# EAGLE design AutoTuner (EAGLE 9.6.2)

## Sheet 1 of 4: mcu
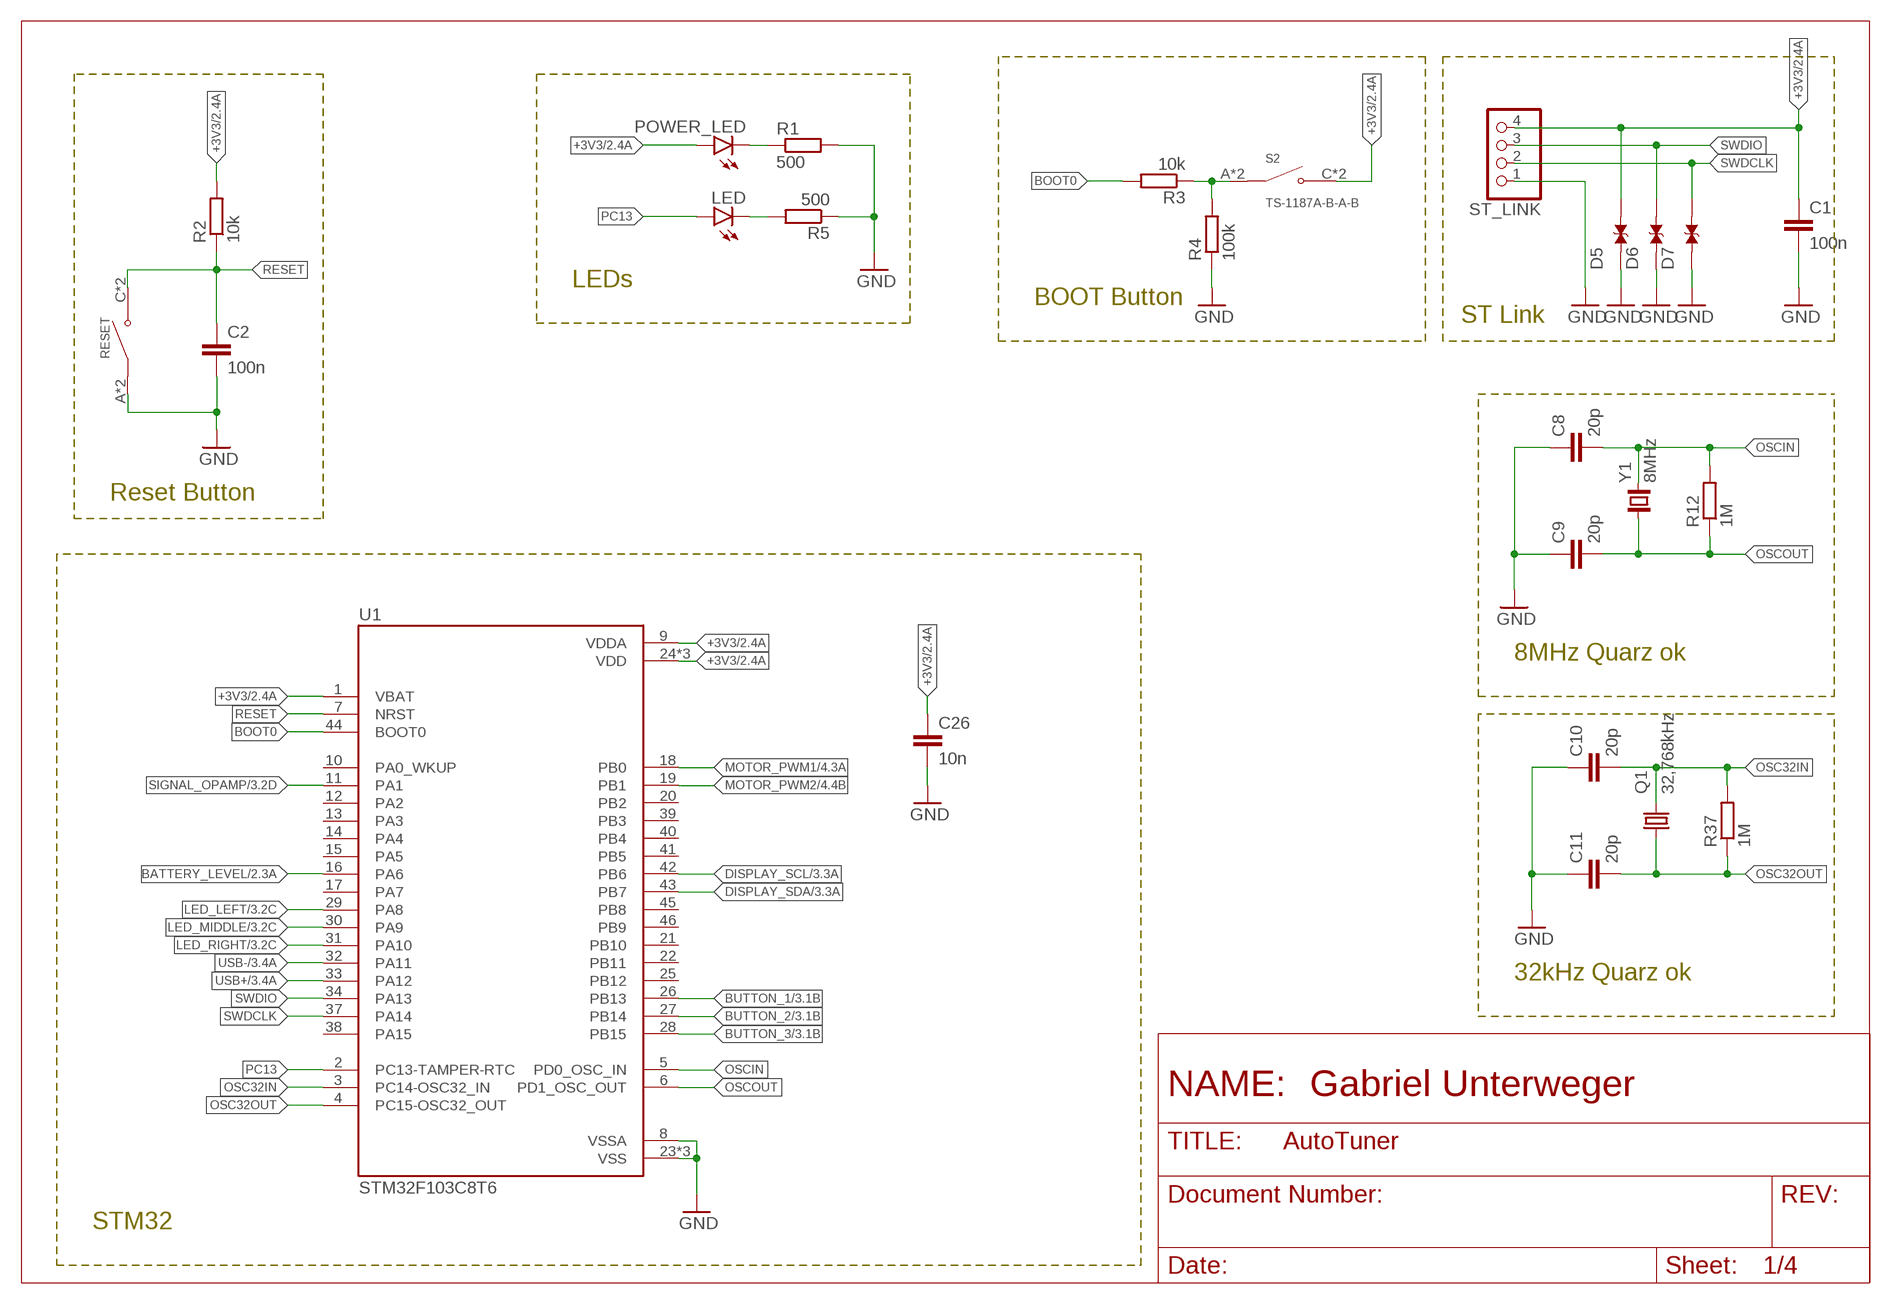
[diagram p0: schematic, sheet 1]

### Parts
C1  100n  C-EUC0805  [C0805]
C2  100n  C-EUC0805  [C0805]
C8  20p  C-EUC0805  [C0805]
C9  20p  C-EUC0805  [C0805]
C10  20p  C-EUC0805  [C0805]
C11  20p  C-EUC0805  [C0805]
C26  10n  C-EUC0805  [C0805]
D5  TESD5V0L1UC_RJG  [DIO_TESD5V0L1UC_RJG]
D6  TESD5V0L1UC_RJG  [DIO_TESD5V0L1UC_RJG]
D7  TESD5V0L1UC_RJG  [DIO_TESD5V0L1UC_RJG]
LED  LEDCHIPLED_0805  [CHIPLED_0805]
POWER_LED  LEDCHIPLED_0805  [CHIPLED_0805]
Q1  32,768kHz  KX-327-NHF  [3.2X1.5]
R1  500  R-EU_R0805  [R0805]
R2  10k  R-EU_R0805  [R0805]
R3  10k  R-EU_R0805  [R0805]
R4  100k  R-EU_R0805  [R0805]
R5  500  R-EU_R0805  [R0805]
R12  1M  R-EU_R0805  [R0805]
R37  1M  R-EU_R0805  [R0805]
RESET  TS-1187A-B-A-B  [SW_TS-1187A-B-A-B]
S2  TS-1187A-B-A-B  [SW_TS-1187A-B-A-B]
ST_LINK  PINHD-1X4  [1X04]
U1  STM32F103C8T6  [QFP50P900X900X160-48N]
Y1  8MHz  CRYSTAL_NX5032GA  [CRYSTAL_2-SMD-5X3]

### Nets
+3V3: C1.1 C26.1 D5.2 POWER_LED.A R2.2 S2.C(NO) S2.D(NO) ST_LINK.4 U1.1(VBAT) U1.9(VDDA) U1.24(VDD) U1.36(VDD) U1.48(VDD) ; also sheet 2,3,4
BATTERY_LEVEL: U1.16(PA6) ; also sheet 2
BOOT0: R3.2 U1.44(BOOT0)
BUTTON_1: U1.26(PB13) ; also sheet 3
BUTTON_2: U1.27(PB14) ; also sheet 3
BUTTON_3: U1.28(PB15) ; also sheet 3
DISPLAY_SCL: U1.42(PB6) ; also sheet 3
DISPLAY_SDA: U1.43(PB7) ; also sheet 3
GND: C1.2 C2.2 C8.1 C9.1 C10.1 C11.1 C26.2 D5.1 D6.1 D7.1 R1.2 R4.1 R5.1 RESET.A(COM) RESET.B(COM) ST_LINK.1 U1.8(VSSA) U1.23(VSS) U1.35(VSS) U1.47(VSS) ; also sheet 2,3,4
LED_LEFT: U1.29(PA8) ; also sheet 3
LED_MIDDLE: U1.30(PA9) ; also sheet 3
LED_RIGHT: U1.31(PA10) ; also sheet 3
MOTOR_PWM1: U1.18(PB0) ; also sheet 4
MOTOR_PWM2: U1.19(PB1) ; also sheet 4
N$2: LED.C R5.2
N$3: POWER_LED.C R1.1
N$5: R3.1 R4.2 S2.A(COM) S2.B(COM)
OSC32IN: C10.2 Q1.2 R37.2 U1.3(PC14-OSC32_IN)
OSC32OUT: C11.2 Q1.1 R37.1 U1.4(PC15-OSC32_OUT)
OSCIN: C8.2 R12.2 U1.5(PD0_OSC_IN) Y1.2
OSCOUT: C9.2 R12.1 U1.6(PD1_OSC_OUT) Y1.1
PC13: LED.A U1.2(PC13-TAMPER-RTC)
RESET: C2.1 R2.1 RESET.C(NO) RESET.D(NO) U1.7(NRST)
SIGNAL_OPAMP: U1.11(PA1) ; also sheet 3,4
SWDCLK: D7.2 ST_LINK.2 U1.37(PA14)
SWDIO: D6.2 ST_LINK.3 U1.34(PA13)
USB+: U1.33(PA12) ; also sheet 3
USB-: U1.32(PA11) ; also sheet 3
Unconnected: U1.10(PA0_WKUP) U1.12(PA2) U1.13(PA3) U1.14(PA4) U1.15(PA5) U1.17(PA7) U1.20(PB2) U1.21(PB10) U1.22(PB11) U1.25(PB12) U1.38(PA15) U1.39(PB3) U1.40(PB4) U1.41(PB5) U1.45(PB8) U1.46(PB9)

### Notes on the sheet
- LEDs
- BOOT Button
- ST Link
- Reset Button
- 8MHz Quarz ok
- 32kHz Quarz ok
- STM32

## Sheet 2 of 4: battery / voltage converter
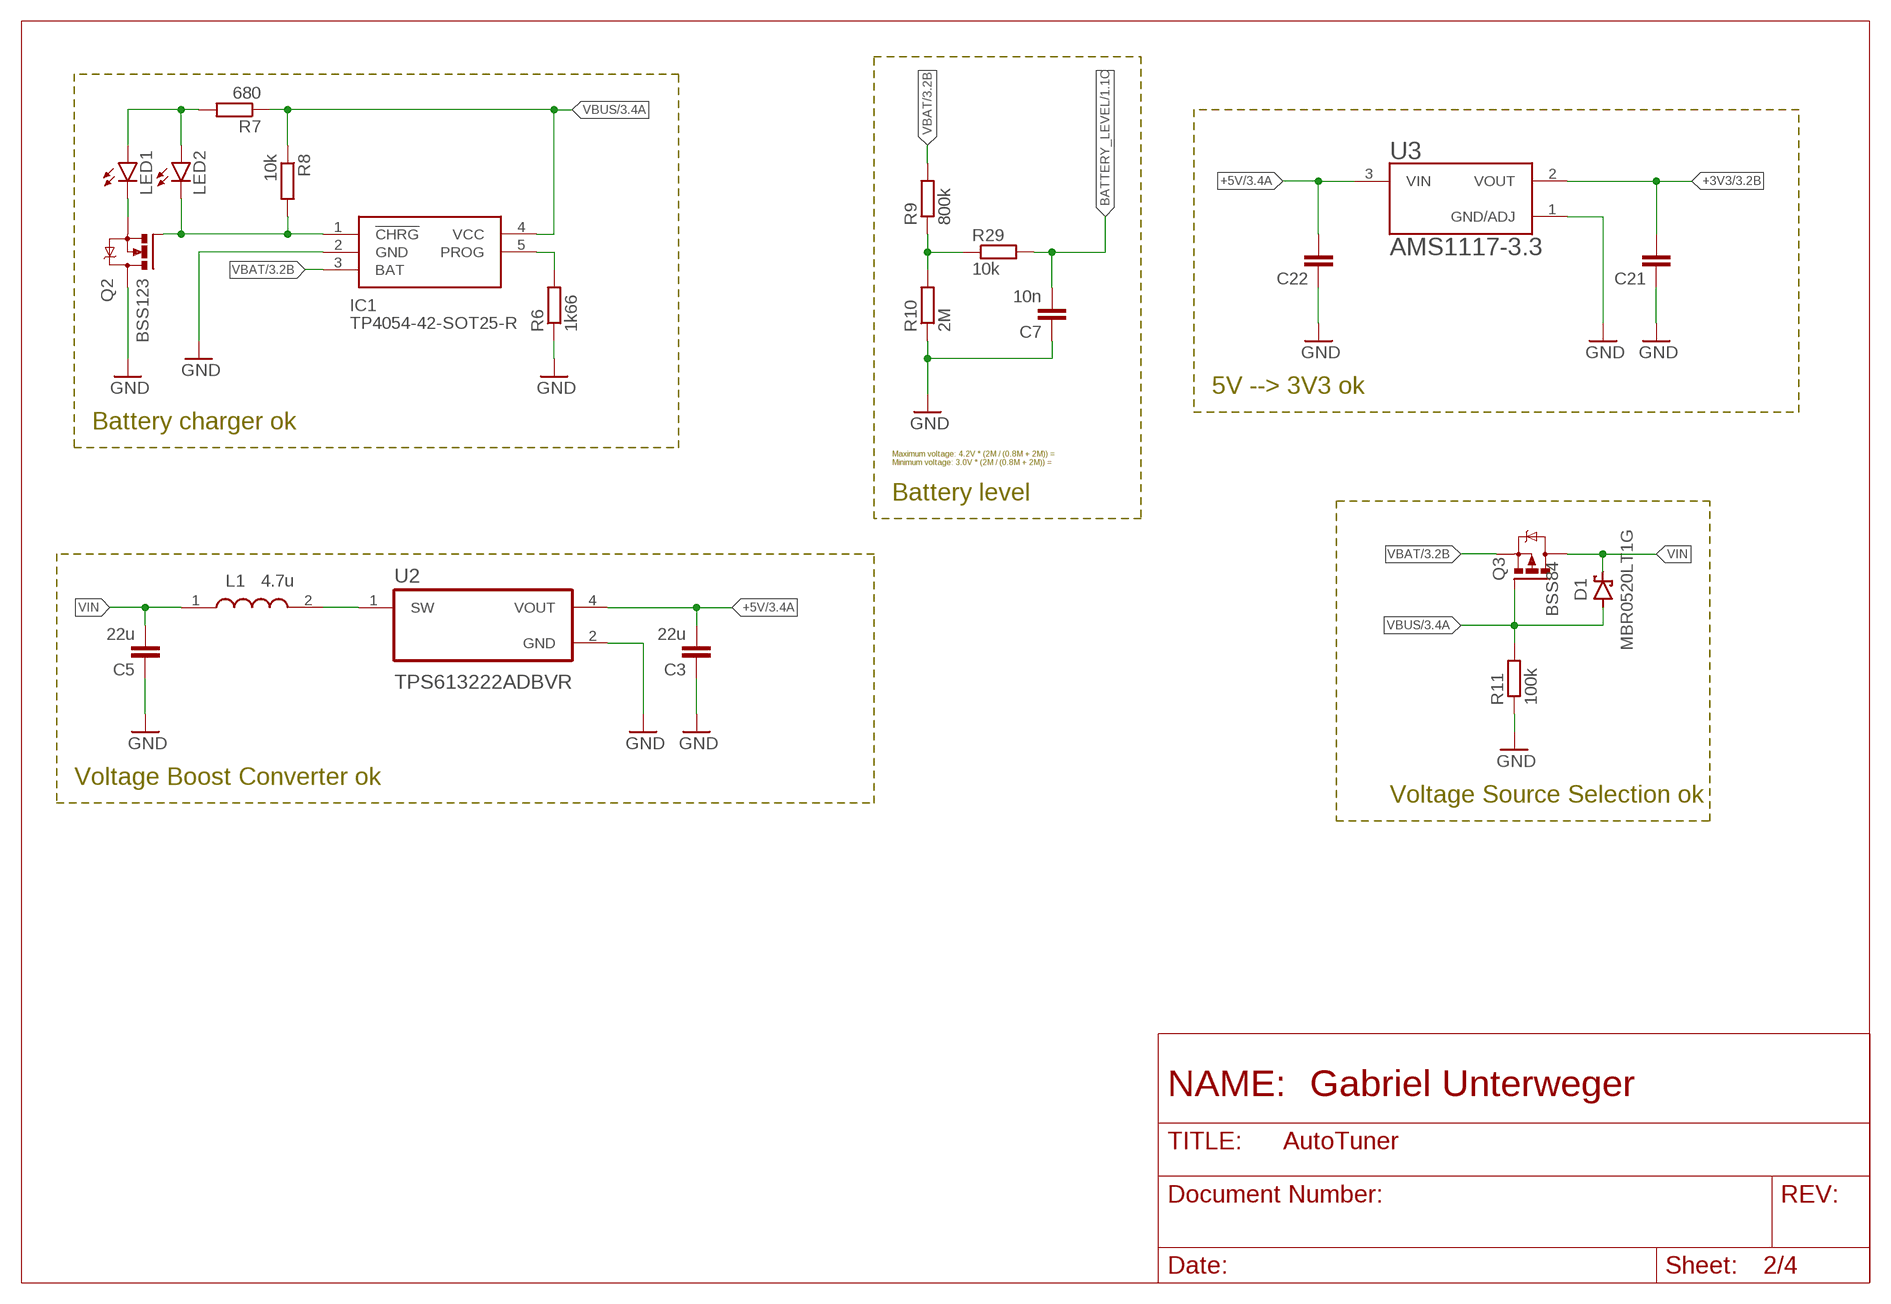
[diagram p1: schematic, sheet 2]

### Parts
C3  22u  C-EUC0805  [C0805]
C5  22u  C-EUC0805  [C0805]
C7  10n  C-EUC0805  [C0805]
C21  C-EUC0805  [C0805]
C22  C-EUC0805  [C0805]
D1  MBR0520LT1G  SCHOTTKY_MBR0520LT1GDO-219  [SODFL3718X115]
IC1  TP4054-42-SOT25-R  [SOT95P280X100-5N]
L1  4.7u  DFE252012P-4R7M=P2  [DFE2HCAH1R0MJ0L]
LED1  LEDCHIPLED_0805  [CHIPLED_0805]
LED2  LEDCHIPLED_0805  [CHIPLED_0805]
Q2  BSS123  NMOSFET_BSS123_SOT23-GSD  [SOT23]
Q3  BSS84  PMOSFET_BSS84_SOT23-GSD  [SOT23]
R6  1k66  R-EU_R0805  [R0805]
R7  680  R-EU_R0805  [R0805]
R8  10k  R-EU_R0805  [R0805]
R9  800k  R-EU_R0805  [R0805]
R10  2M  R-EU_R0805  [R0805]
R11  100k  R-EU_R0805  [R0805]
R29  10k  R-EU_R0805  [R0805]
U2  TPS613222ADBVR  [SOT95P280X145-5N]
U3  AMS1117-3.3  [SOT229P700X180-4N]

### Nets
+3V3: C21.2 U3.2(VOUT) ; also sheet 1,3,4
+5V: C3.2 C22.2 U2.4(VOUT) U3.3(VIN) ; also sheet 3
BATTERY_LEVEL: C7.2 R29.2 ; also sheet 1
GND: C3.1 C5.1 C7.1 C21.1 C22.1 IC1.2(GND) Q2.3(D) R6.1 R10.1 R11.1 U2.2(GND) U3.1(GND/ADJ) ; also sheet 1,3,4
N$1: L1.2 U2.1(SW)
N$4: R9.1 R10.2 R29.1
N$8: IC1.5(PROG) R6.2
N$9: IC1.1(!CHRG) LED2.C Q2.1(G) R8.2
N$11: LED1.A LED2.A R7.2
N$12: LED1.C Q2.2(S)
VBAT: IC1.3(BAT) Q3.2(S) R9.2 ; also sheet 3,4
VBUS: D1.2(A) IC1.4(VCC) Q3.1(G) R7.1 R8.1 R11.2 ; also sheet 3
VIN: C5.2 D1.1(C) L1.1 Q3.3(D)

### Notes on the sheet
- 5V --> 3V3 ok
- Battery charger ok
- Maximum voltage: 4.2V * (2M / (0.8M + 2M)) =
  Minimum voltage: 3.0V * (2M / (0.8M + 2M)) =
- Battery level
- Voltage Boost Converter ok
- Voltage Source Selection ok

## Sheet 3 of 4: I/O
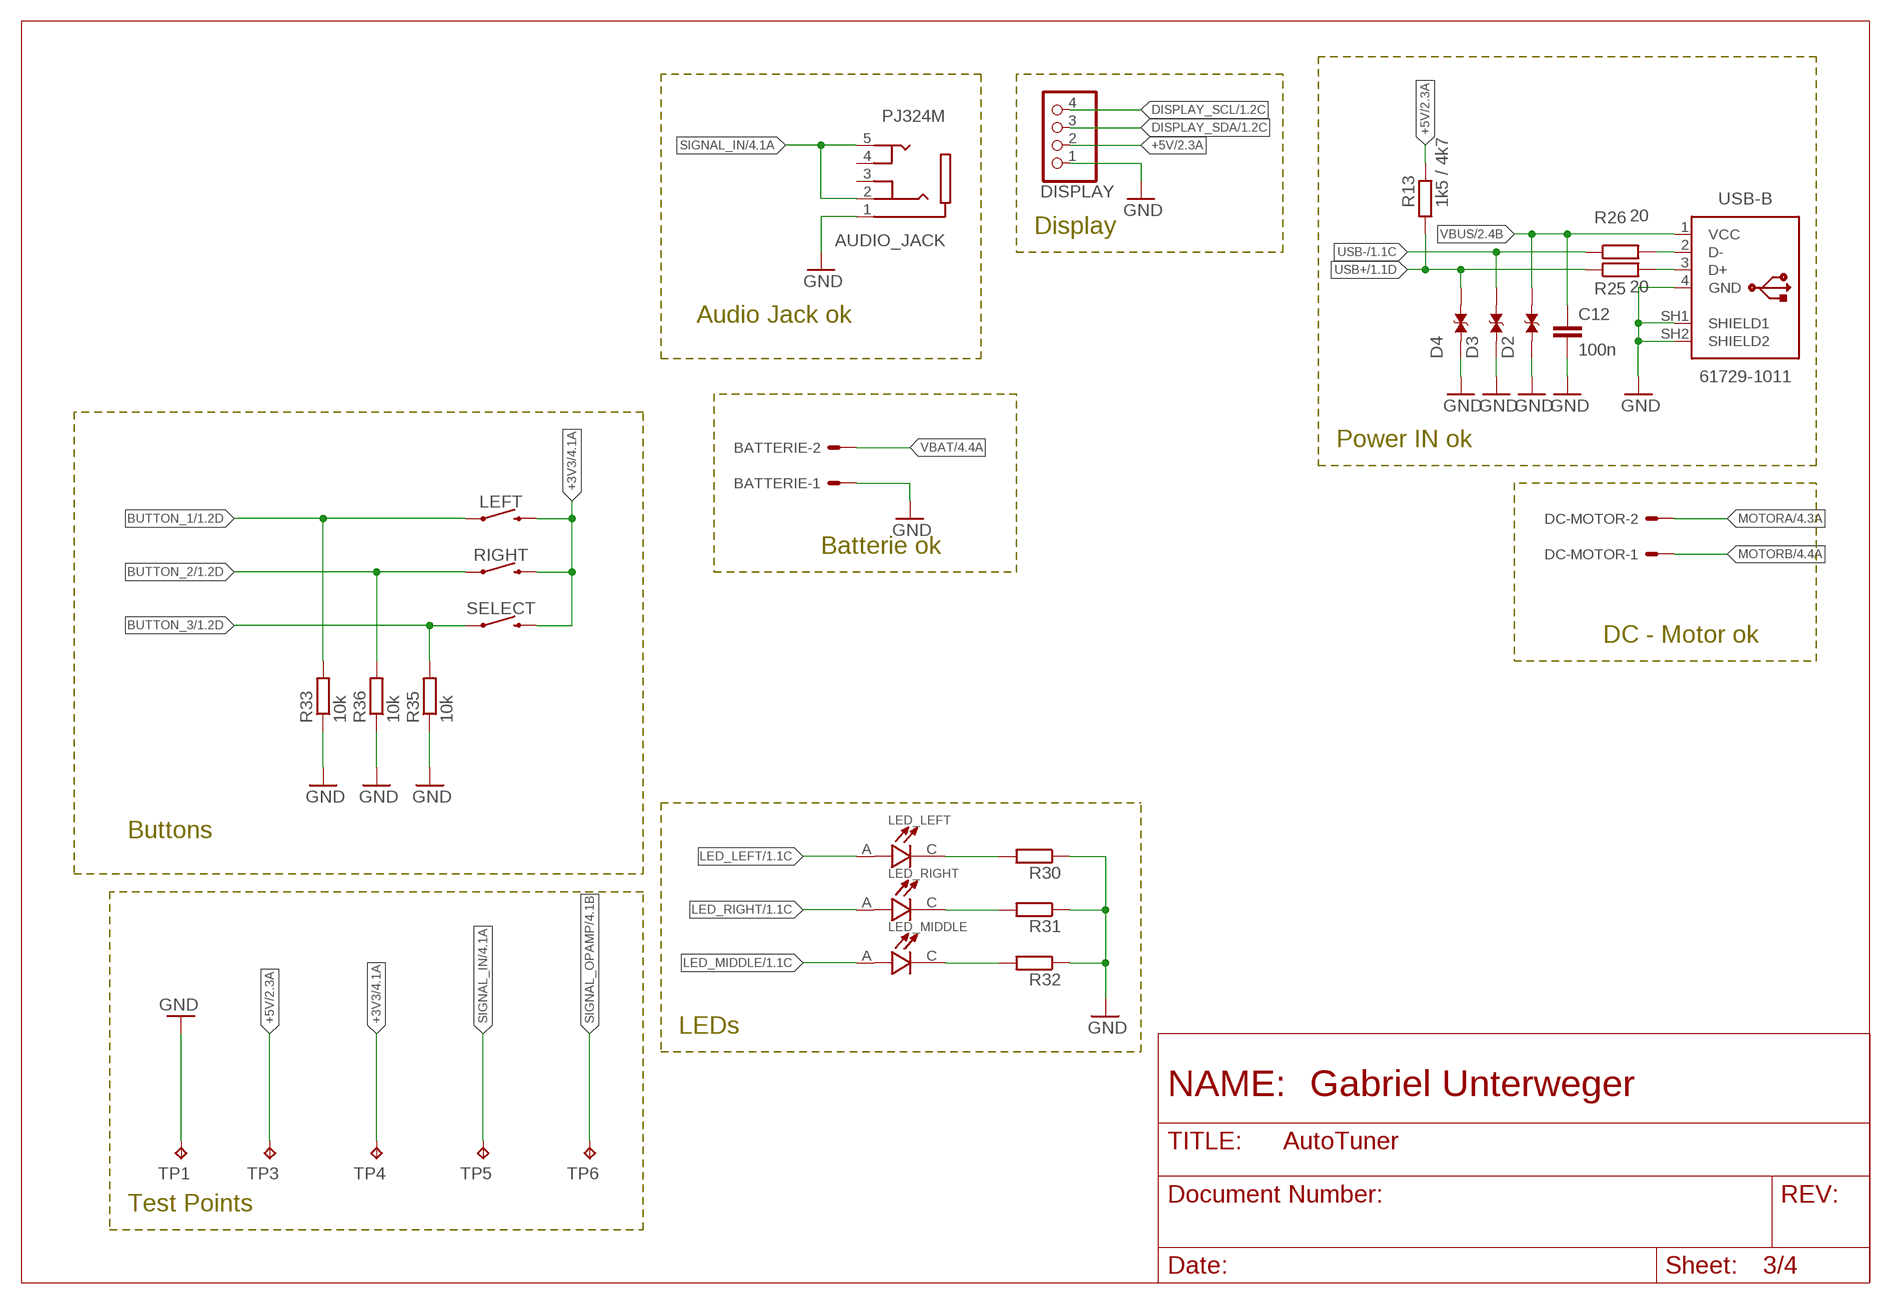
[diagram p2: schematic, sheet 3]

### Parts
AUDIO_JACK  PJ324M  [WENZHOU_PJ324M]
BATTERIE  22-27-2021-02  [6410-02]
C12  100n  C-EUC0805  [C0805]
D2  TESD5V0L1UC_RJG  [DIO_TESD5V0L1UC_RJG]
D3  TESD5V0L1UC_RJG  [DIO_TESD5V0L1UC_RJG]
D4  TESD5V0L1UC_RJG  [DIO_TESD5V0L1UC_RJG]
DC-MOTOR  22-27-2021-02  [6410-02]
DISPLAY  PINHD-1X4  [1X04]
LED_LEFT  L-53GD  [LEDRD254W50D500H1060]
LED_MIDDLE  L-53GD  [LEDRD254W50D500H1060]
LED_RIGHT  L-53GD  [LEDRD254W50D500H1060]
LEFT  MOMENTARY-SWITCH-SPST-PTH-12MM  [TACTILE_SWITCH_PTH_12MM]
R13  1k5 / 4k7  R-EU_R0805  [R0805]
R25  20  R-EU_R0805  [R0805]
R26  20  R-EU_R0805  [R0805]
R30  R-EU_R0805  [R0805]
R31  R-EU_R0805  [R0805]
R32  R-EU_R0805  [R0805]
R33  10k  R-EU_R0805  [R0805]
R35  10k  R-EU_R0805  [R0805]
R36  10k  R-EU_R0805  [R0805]
RIGHT  MOMENTARY-SWITCH-SPST-PTH-12MM  [TACTILE_SWITCH_PTH_12MM]
SELECT  MOMENTARY-SWITCH-SPST-PTH-12MM  [TACTILE_SWITCH_PTH_12MM]
TP1  TPB1,27  [B1,27]
TP3  TPB1,27  [B1,27]
TP4  TPB1,27  [B1,27]
TP5  TPB1,27  [B1,27]
TP6  TPB1,27  [B1,27]
USB-B  61729-1011  [61729-1011BLF]

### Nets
+3V3: LEFT.3 RIGHT.3 SELECT.3 TP4.TP ; also sheet 1,2,4
+5V: DISPLAY.2 R13.2 TP3.TP ; also sheet 2
BUTTON_1: LEFT.1 R33.2 ; also sheet 1
BUTTON_2: R36.2 RIGHT.1 ; also sheet 1
BUTTON_3: R35.2 SELECT.1 ; also sheet 1
DISPLAY_SCL: DISPLAY.4 ; also sheet 1
DISPLAY_SDA: DISPLAY.3 ; also sheet 1
GND: AUDIO_JACK.1(SLEEVE) BATTERIE.1 C12.2 D2.1 D3.1 D4.1 DISPLAY.1 R30.1 R31.1 R32.1 R33.1 R35.1 R36.1 TP1.TP USB-B.4(GND) USB-B.SH1(SHIELD1) USB-B.SH2(SHIELD2) ; also sheet 1,2,4
LED_LEFT: LED_LEFT.A ; also sheet 1
LED_MIDDLE: LED_MIDDLE.A ; also sheet 1
LED_RIGHT: LED_RIGHT.A ; also sheet 1
MOTORA: DC-MOTOR.2 ; also sheet 4
MOTORB: DC-MOTOR.1 ; also sheet 4
N$19: LED_LEFT.C R30.2
N$20: LED_RIGHT.C R31.2
N$23: LED_MIDDLE.C R32.2
N$29: R25.2 USB-B.3(D+)
N$30: R26.2 USB-B.2(D-)
SIGNAL_IN: AUDIO_JACK.2(RING_1) AUDIO_JACK.5(TIP_2) TP5.TP ; also sheet 4
SIGNAL_OPAMP: TP6.TP ; also sheet 1,4
USB+: D4.2 R13.1 R25.1 ; also sheet 1
USB-: D3.2 R26.1 ; also sheet 1
VBAT: BATTERIE.2 ; also sheet 2,4
VBUS: C12.1 D2.2 USB-B.1(VCC) ; also sheet 2
Unconnected: AUDIO_JACK.3(RING_2) AUDIO_JACK.4(TIP_1)

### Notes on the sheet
- Display
- Audio Jack ok
- Power IN ok
- Batterie ok
- DC - Motor ok
- Buttons
- LEDs
- Test Points

## Sheet 4 of 4: Motor Steuerung / Signal Verarbeitung
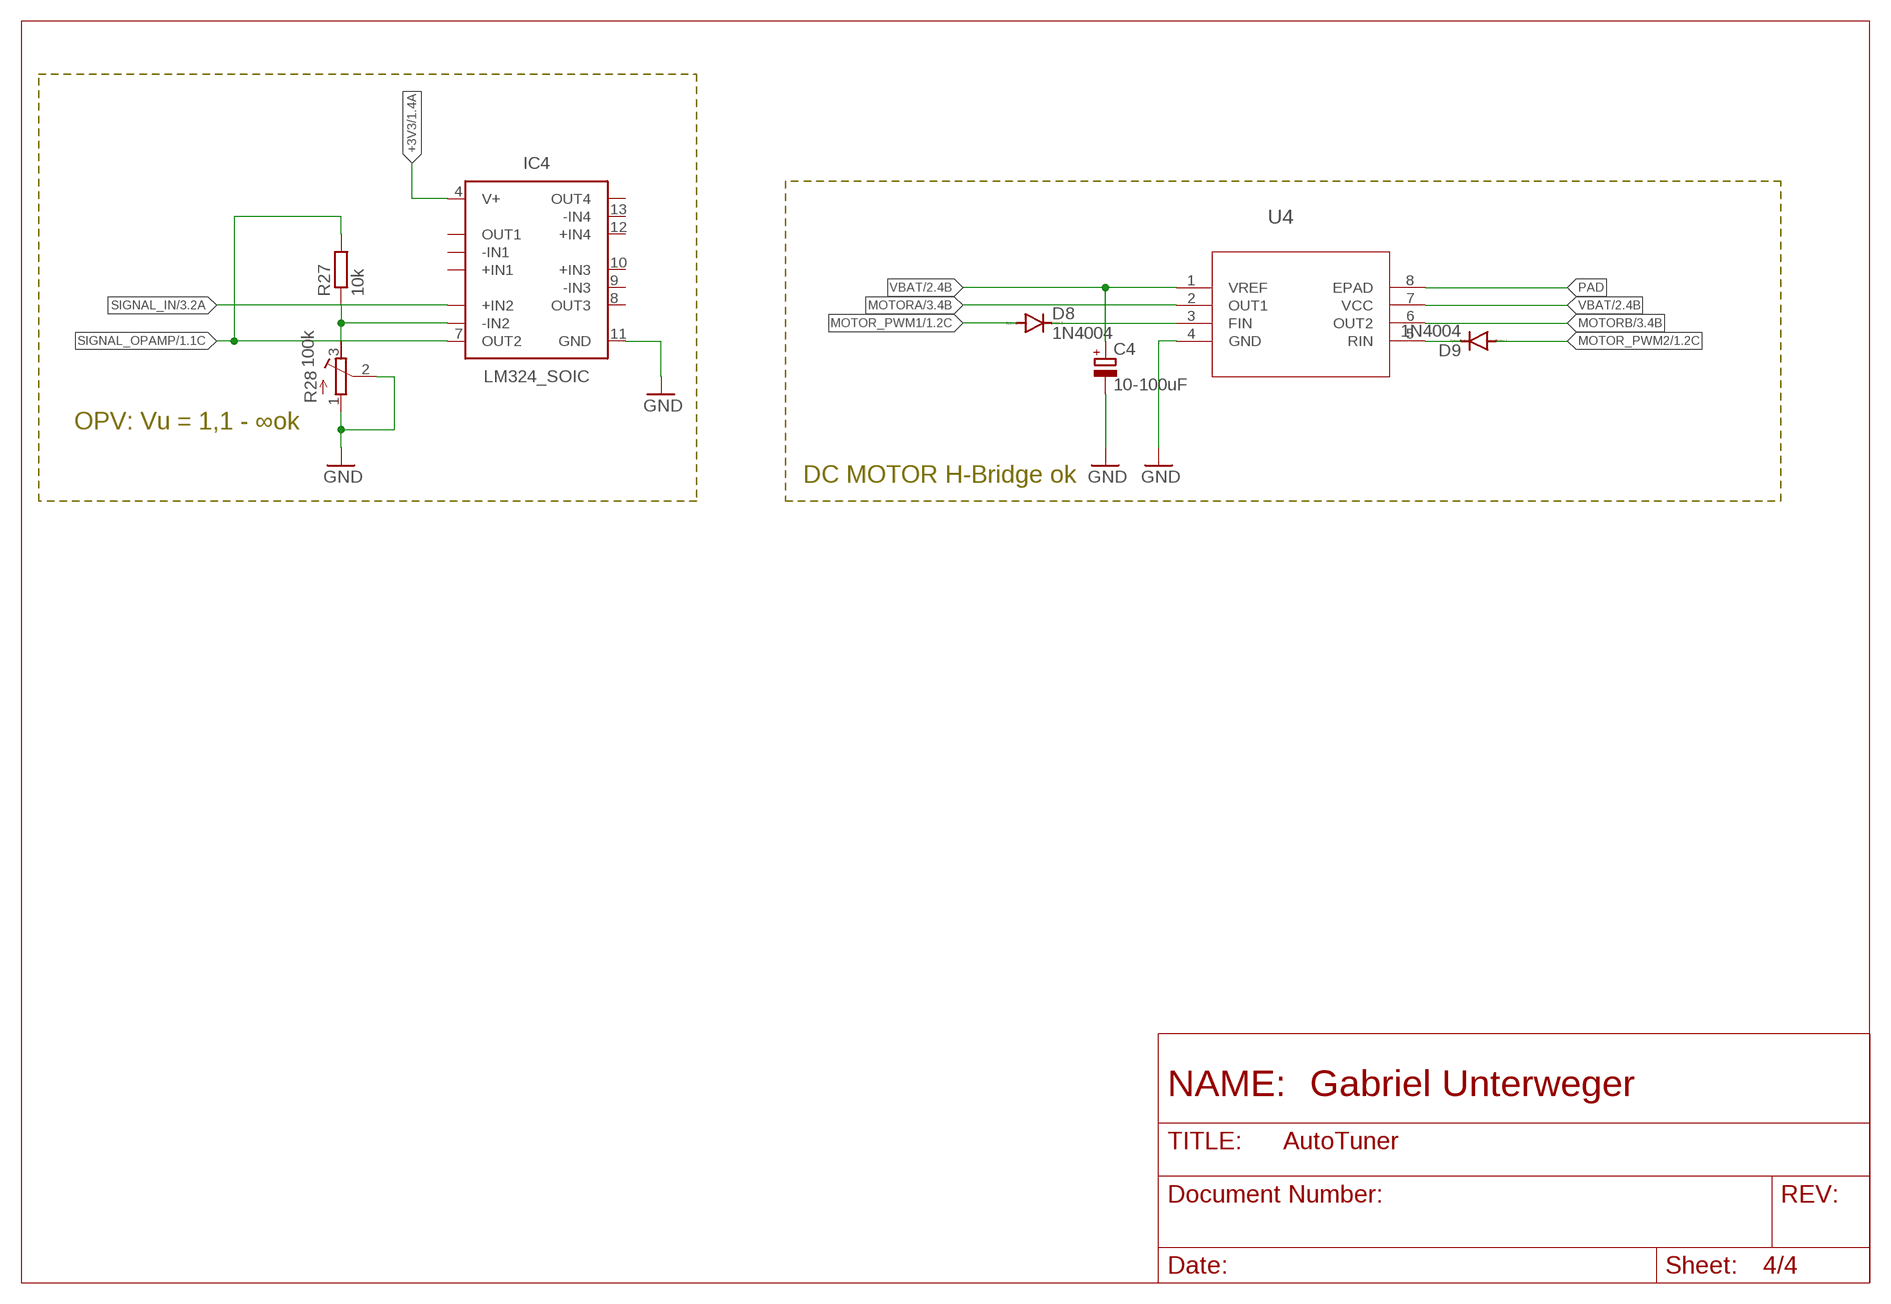
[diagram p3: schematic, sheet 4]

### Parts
C4  10-100uF  CPOL-EUB45181A  [B45181A]
D8  1N4004  [DO41-10]
D9  1N4004  [DO41-10]
IC4  LM324_SOIC  [SOIC127P600X175-14N]
R27  10k  R-EU_R0805  [R0805]
R28  100k  R-TRIMM3296X  [RTRIM3296X]
U4  BD6222HFP-TRHRP7_ROM-M  [HRP7_ROM-M]

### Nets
+3V3: IC4.4(V+) ; also sheet 1,2,3
GND: C4.- IC4.11(GND) R28.1(A) R28.2(S) U4.4(GND) ; also sheet 1,2,3
MOTOR_PWM1: D8.A ; also sheet 1
MOTOR_PWM2: D9.A ; also sheet 1
MOTORA: U4.2(OUT1) ; also sheet 3
MOTORB: U4.6(OUT2) ; also sheet 3
N$6: D8.C U4.3(FIN)
N$7: U4.7(VCC)
N$14: D9.C U4.5(RIN)
N$16: IC4.6(-IN2) R27.1 R28.3(E)
PAD: U4.8(EPAD)
SIGNAL_IN: IC4.5(+IN2) ; also sheet 3
SIGNAL_OPAMP: IC4.7(OUT2) R27.2 ; also sheet 1,3
VBAT: C4.+ U4.1(VREF) ; also sheet 2,3
Unconnected: IC4.1(OUT1) IC4.2(-IN1) IC4.3(+IN1) IC4.8(OUT3) IC4.9(-IN3) IC4.10(+IN3) IC4.12(+IN4) IC4.13(-IN4) IC4.14(OUT4)

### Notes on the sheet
- OPV: Vu = 1,1 - ∞ok
- DC MOTOR H-Bridge ok

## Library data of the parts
AUDIO_JACK = PJ324M:PJ324M: Headphone Stereo jack/Audio connector Check availability; AVAILABILITY: Not in stock; CHECK_PRICES: https://www.snapeda.com/parts/PJ324M/Wenzhou+QingPu+Electronics+Co.Ltd/view-part/?ref=eda; DESCRIPTION: Headphone Stereo jack/Audio connector; MF: Wenzhou QingPu Electronics Co.Ltd; MP: PJ324M; PACKAGE: Package; PRICE: None; SNAPEDA_LINK: https://www.snapeda.com/parts/PJ324M/Wenzhou+QingPu+Electronics+Co.Ltd/view-part/?ref=snap
BATTERIE DC-MOTOR = con-molex:22-?-02: CONNECTOR; MF: MOLEX; OC_FARNELL: unknown; OC_NEWARK: unknown
C1-C3 C5 C7-C12 C21 C22 C26 = rcl:C-EU: CAPACITOR, European symbol; SPICEPREFIX: C
C4 = rcl:CPOL-EU: POLARIZED CAPACITOR, European symbol; SPICEPREFIX: C
D1 = Diode:SCHOTTKY_: Schottky Diode - Popular parts; CATEGORY: Diode; DESCRIPTION: DIODE SCHOTTKY 20V 500MA SOD123; LCSC_PART: C191023; MANUFACTURER: ON Semiconductor; MPN: MBR0520LT1G; SUB-CATEGORY: Schottky
D2-D7 = TESD5V0L1UC_RJG:TESD5V0L1UC_RJG: Check availability; AVAILABILITY: In Stock; CHECK_PRICES: https://www.snapeda.com/parts/TESD5V0L1UC%20RJG/Taiwan+Semiconductor/view-part/?ref=eda; DESCRIPTION: DFN1006L, 5V, 100W, 2pF, ESD Protection Diode & Array; LCSC_PART: C7420372; MF: Taiwan Semiconductor Corporation; MP: TESD5V0L1UC RJG; PACKAGE: DFN1006L Taiwan Semiconductor; PRICE: None; PURCHASE-URL: https://www.snapeda.com/api/url_track_click_mouser/?unipart_id=3789592&manufacturer=Taiwan Semiconductor Corporation&part_name=TESD5V0L1UC RJG&search_term=protection diode; SNAPEDA_LINK: https://www.snapeda.com/parts/TESD5V0L1UC%20RJG/Taiwan+Semiconductor/view-part/?ref=snap
D8 D9 = diode:1N4004: DIODE
DISPLAY ST_LINK = pinhead:PINHD-1X4: PIN HEADER
IC1 = TP4054-42-SOT25-R:TP4054-42-SOT25-R: Standalone Linear Li-ion Battery Charger with Thermal Regulation, SOT-23-5 Source: Datasheet; DESCRIPTION: Standalone Linear Li-ion Battery Charger with Thermal Regulation, SOT-23-5; HEIGHT: 1mm; LCSC_PART: C32574; MANUFACTURER_NAME: TOP POWER; MANUFACTURER_PART_NUMBER: TP4054-42-SOT25-R
IC4 = IC_Linear:LM324: Quad-Operational Amplifiers Reference Datasheet; CATEGORY: Operational Amplifiers; DESCRIPTION: Quad-Operational Amplifiers; LCSC_PART: C71035; MANUFACTURER: Generic; MPN: Generic; SERIES: LM324; SUB-CATEGORY: Amplifier ICs; TYPE: Op Amps - Operational Amplifiers
L1 = DFE252012P-4R7M=P2:DFE252012P-4R7M=P2: Toko DFE252012P Series Shielded Wire-wound SMD Inductor with a Powered Iron Core, 4.7 uH Wire-Wound 2.2A Idc; ARROW_PART_NUMBER: DFE252012P-4R7M=P2; ARROW_PRICE-STOCK: https://www.arrow.com/en/products/dfe252012p-4r7mp2/murata-manufacturing?region=europe; DESCRIPTION: Toko DFE252012P Series Shielded Wire-wound SMD Inductor with a Powered Iron Core, 4.7 uH Wire-Wound 2.2A Idc; HEIGHT: 1.2mm; LCSC_PART: C391306; MANUFACTURER_NAME: Murata Electronics; MANUFACTURER_PART_NUMBER: DFE252012P-4R7M=P2; MOUSER_PART_NUMBER: 81-DFE252012P-4R7MP2; MOUSER_PRICE-STOCK: https://www.mouser.co.uk/ProductDetail/Murata-Electronics/DFE252012P-4R7M%3dP2?qs=KuGPmAKtFKVp8Hnp6vDIBg%3D%3D
LED LED1 LED2 POWER_LED = led:LED: LED
LED_LEFT LED_MIDDLE LED_RIGHT = L-53GD:L-53GD: LED; 5mm; green; 5-32mcd; 60°; Front: convex Check availability; AVAILABILITY: In Stock; CHECK_PRICES: https://www.snapeda.com/parts/L-53GD/Kingbright/view-part/?ref=eda; DESCRIPTION: LED; 5mm; green; 5-32mcd; 60°; Front: convex; MF: Kingbright; MP: L-53GD; PACKAGE: CDIP-28 Kingbright; PRICE: None; PURCHASE-URL: https://www.snapeda.com/api/url_track_click_mouser/?unipart_id=525636&manufacturer=Kingbright&part_name=L-53GD&search_term=led, 5mm; SNAPEDA_LINK: https://www.snapeda.com/parts/L-53GD/Kingbright/view-part/?ref=snap
LEFT RIGHT SELECT = SparkFun-Switches:MOMENTARY-SWITCH-SPST: Momentary Switch (Pushbutton) - SPST; PROD_ID: SWCH-09185; SF_SKU: COM-09190
Q1 = crystal-geyer_V1_0:KX-327; LCSC_PART: C32346
Q2 = Transistor:NMOSFET_: N-Channel MOSFET - Popular parts; CATEGORY: Transistor; DESCRIPTION: MOSFET N-CH 100V 0.17A SOT-23; DRAIN_CURRENT: 170mA; LCSC_PART: C20917; MANUFACTURER: ON Semiconductor; MPN: BSS123L; OPERATING_TEMP: -55°C ~ 150°C; PART_STATUS: Active; ROHS_COMPLIANT: Yes; SUB-CATEGORY: MOSFET; THERMALLOSS: 360mW; TYPE: N-Channel
Q3 = Transistor:PMOSFET_: P-Channel MOSFET - Popular parts; CATEGORY: Transistor; DESCRIPTION: MOSFET P-CH 50V 130MA SOT-23; DRAIN_CURRENT: 130mA; LCSC_PARTS: C10487; MANUFACTURER: ON Semiconductor; MPN: BSS84; OPERATING_TEMP: -55°C ~ 150°C; PART_STATUS: Active; ROHS_COMPLIANT: Yes; SUB-CATEGORY: MOSFET; THERMALLOSS: 360mW; TYPE: P-Channel
R1-R13 R25-R27 R29-R33 R35-R37 = rcl:R-EU_: RESISTOR, European symbol; SPICEPREFIX: R
R28 = rcl:R-TRIMM: Trimm resistor; SPICEMODEL: X; SPICEPREFIXL: POT
RESET S2 = TS-1187A-B-A-B:TS-1187A-B-A-B: SPST 50mA @ 12VDC Top Actuated Round Button 160gf SMD Tactile Switches RoHS Check availability; AVAILABILITY: Not in stock; DESCRIPTION: TS-1187A-B-A-B XKB Connectivity; LCSC_PART: C318884; MF: XKB Industrial Precision; MP: TS-1187A-B-A-B; PACKAGE: Package; PRICE: None
TP1 TP3-TP6 = testpad:TP: Test pad
U1 = STM32F103C8T6:STM32F103C8T6: Mainstream Performance line, ARM Cortex-M3 MCU with 64 Kbytes Flash, 72 MHz CPU, motor control, USB and CAN Check availability; AVAILABILITY: In Stock; CHECK_PRICES: https://www.snapeda.com/parts/STM32F103C8T6/STMicroelectronics/view-part/?ref=eda; DESCRIPTION: ARM® Cortex®-M3 STM32F1 Microcontroller IC 32-Bit 72MHz 64KB (64K x 8) FLASH 48-LQFP (7x7); LCSC_PART: C8734; MF: STMicroelectronics; MP: STM32F103C8T6; PACKAGE: LQFP-48 STMicroelectronics; PRICE: None; PURCHASE-URL: https://www.snapeda.com/api/url_track_click_mouser/?unipart_id=52195&manufacturer=STMicroelectronics&part_name=STM32F103C8T6&search_term=stm32f103c8t6; SNAPEDA_LINK: https://www.snapeda.com/parts/STM32F103C8T6/STMicroelectronics/view-part/?ref=snap
U2 = TPS613222ADBVR:TPS613222ADBVR: Check availability; AVAILABILITY: In Stock; CHECK_PRICES: https://www.snapeda.com/parts/TPS613222ADBVR/Texas+Instruments/view-part/?ref=eda; DESCRIPTION: 6-uA Quiescent Current, 1.8-A Switch Current Boost Converter; LCSC_PART: C2071163; MF: Texas Instruments; MP: TPS613222ADBVR; PACKAGE: SOT-23-5 Texas Instruments; PRICE: None; PURCHASE-URL: https://www.snapeda.com/api/url_track_click_mouser/?unipart_id=2771858&manufacturer=Texas Instruments&part_name=TPS613222ADBVR&search_term=tps613222a; SNAPEDA_LINK: https://www.snapeda.com/parts/TPS613222ADBVR/Texas+Instruments/view-part/?ref=snap
U3 = AMS1117-3.3:AMS1117-3.3: Check availability; AVAILABILITY: Not in stock; CHECK_PRICES: https://www.snapeda.com/parts/AMS1117-3.3/Advanced+Monolithic+Systems/view-part/?ref=eda; DESCRIPTION: Sot223/Pkg 1-Amp 3.3-Volt Low Drop Out Voltage Regulatator; LCSC_PART: C6186; MF: Advanced Monolithic Systems; MP: AMS1117-3.3; PACKAGE: SOT-223 Seeed Technology; PRICE: None; SNAPEDA_LINK: https://www.snapeda.com/parts/AMS1117-3.3/Advanced+Monolithic+Systems/view-part/?ref=snap
U4 = H-Brücke_BD622HFP-TR02:BD6222HFP-TR; COPYRIGHT: Copyright (C) 2022 Ultra Librarian. All rights reserved.; MANUFACTURER_PART_NUMBER: BD6222HFP-TR; MFR_NAME: ROHM Semiconductor
USB-B = Connector_USB:61729-1011: USB(2.0) Type-B, RCPT, 4POS, THT-R/A Datasheet; CATEGORY: Connector; CONTACTS: 4; CURRENT_RATING: 1A; DESCRIPTION: CONN RCPT USB2.0 TYPEB 4POS R/A; GENDER: Receptacle; MANUFACTURER: Amphenol ICC (FCI); MOUNT_TYPE: R/A; MPN: 61729-1011BLF; OPERATING_TEMP: -55°C to 85°C; PART_STATUS: Active; ROHS_COMPLIANT: RoHS Compliant; SERIES: 61729; SUB-CATEGORY: USB; TYPE: USB-B
Y1 = 52101-101-REV-A_v16:CRYSTAL_NX5032GA: CRYSTAL; LCSC_PART: C115962

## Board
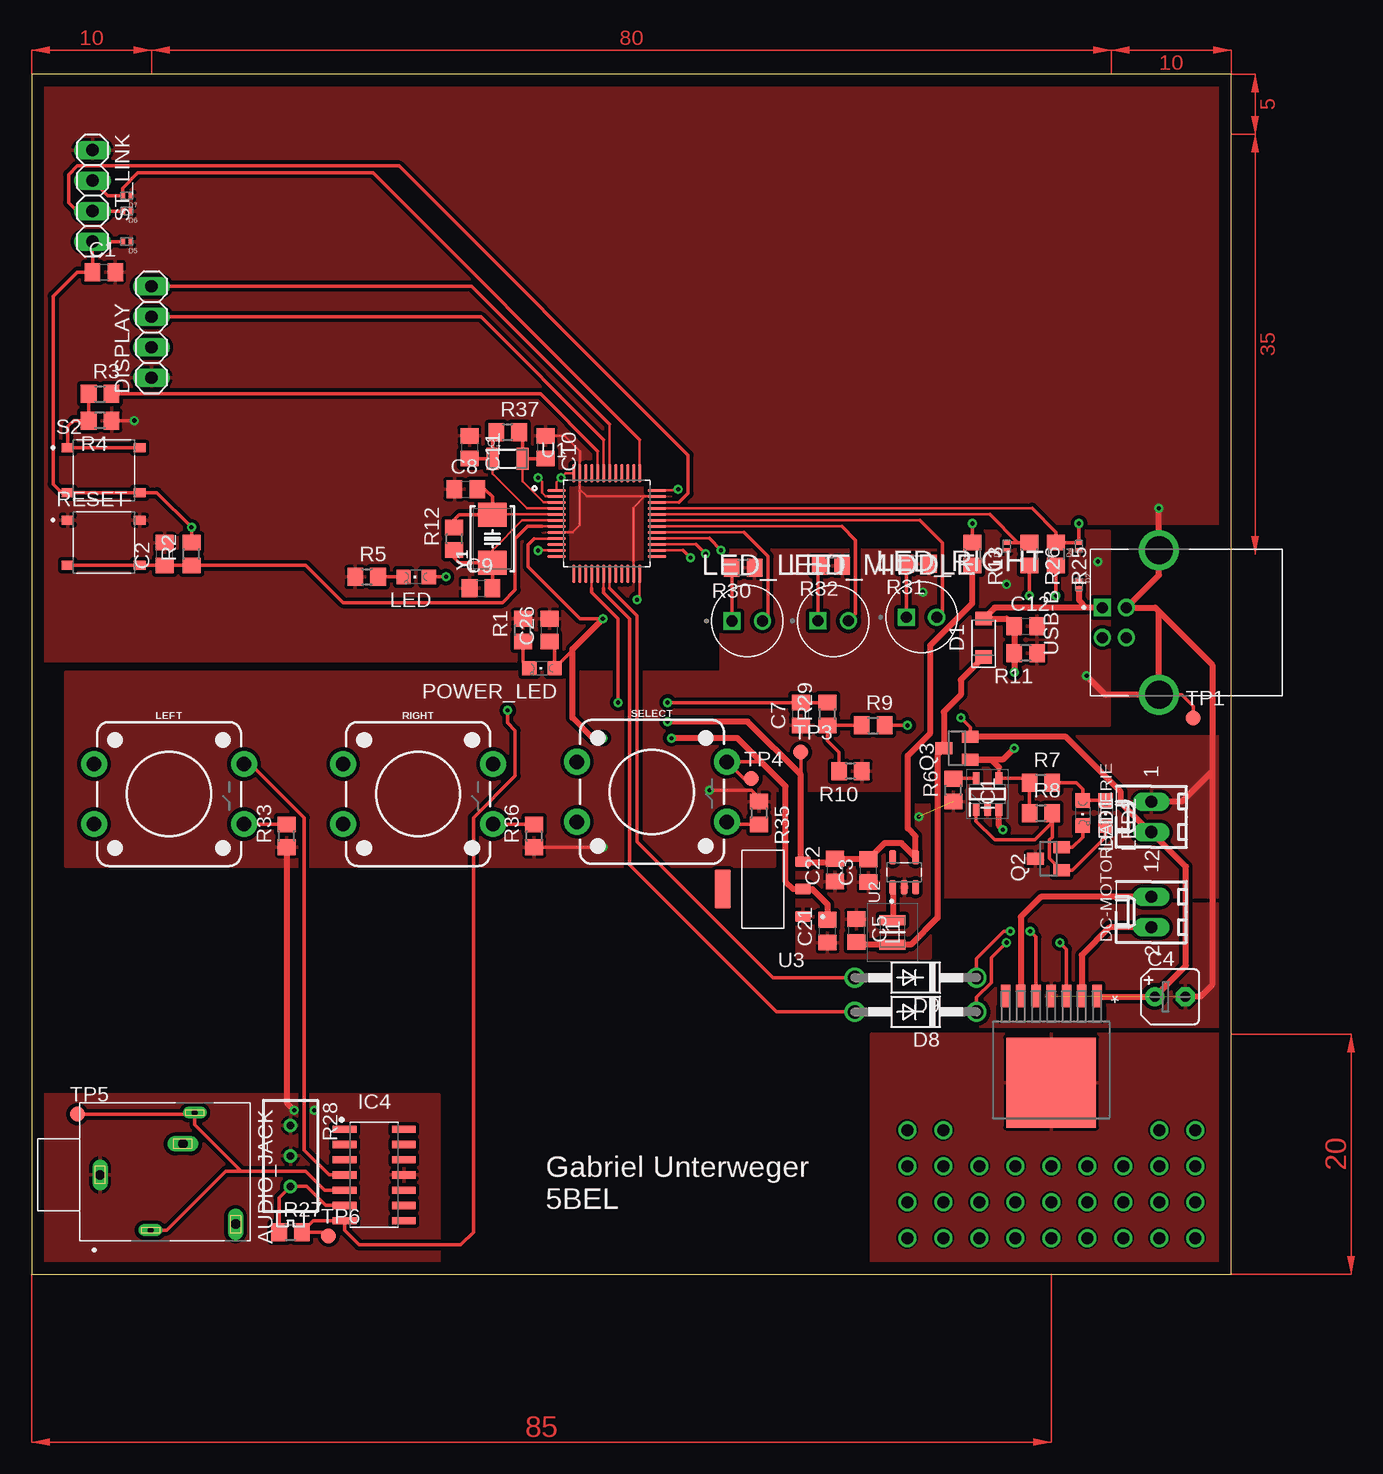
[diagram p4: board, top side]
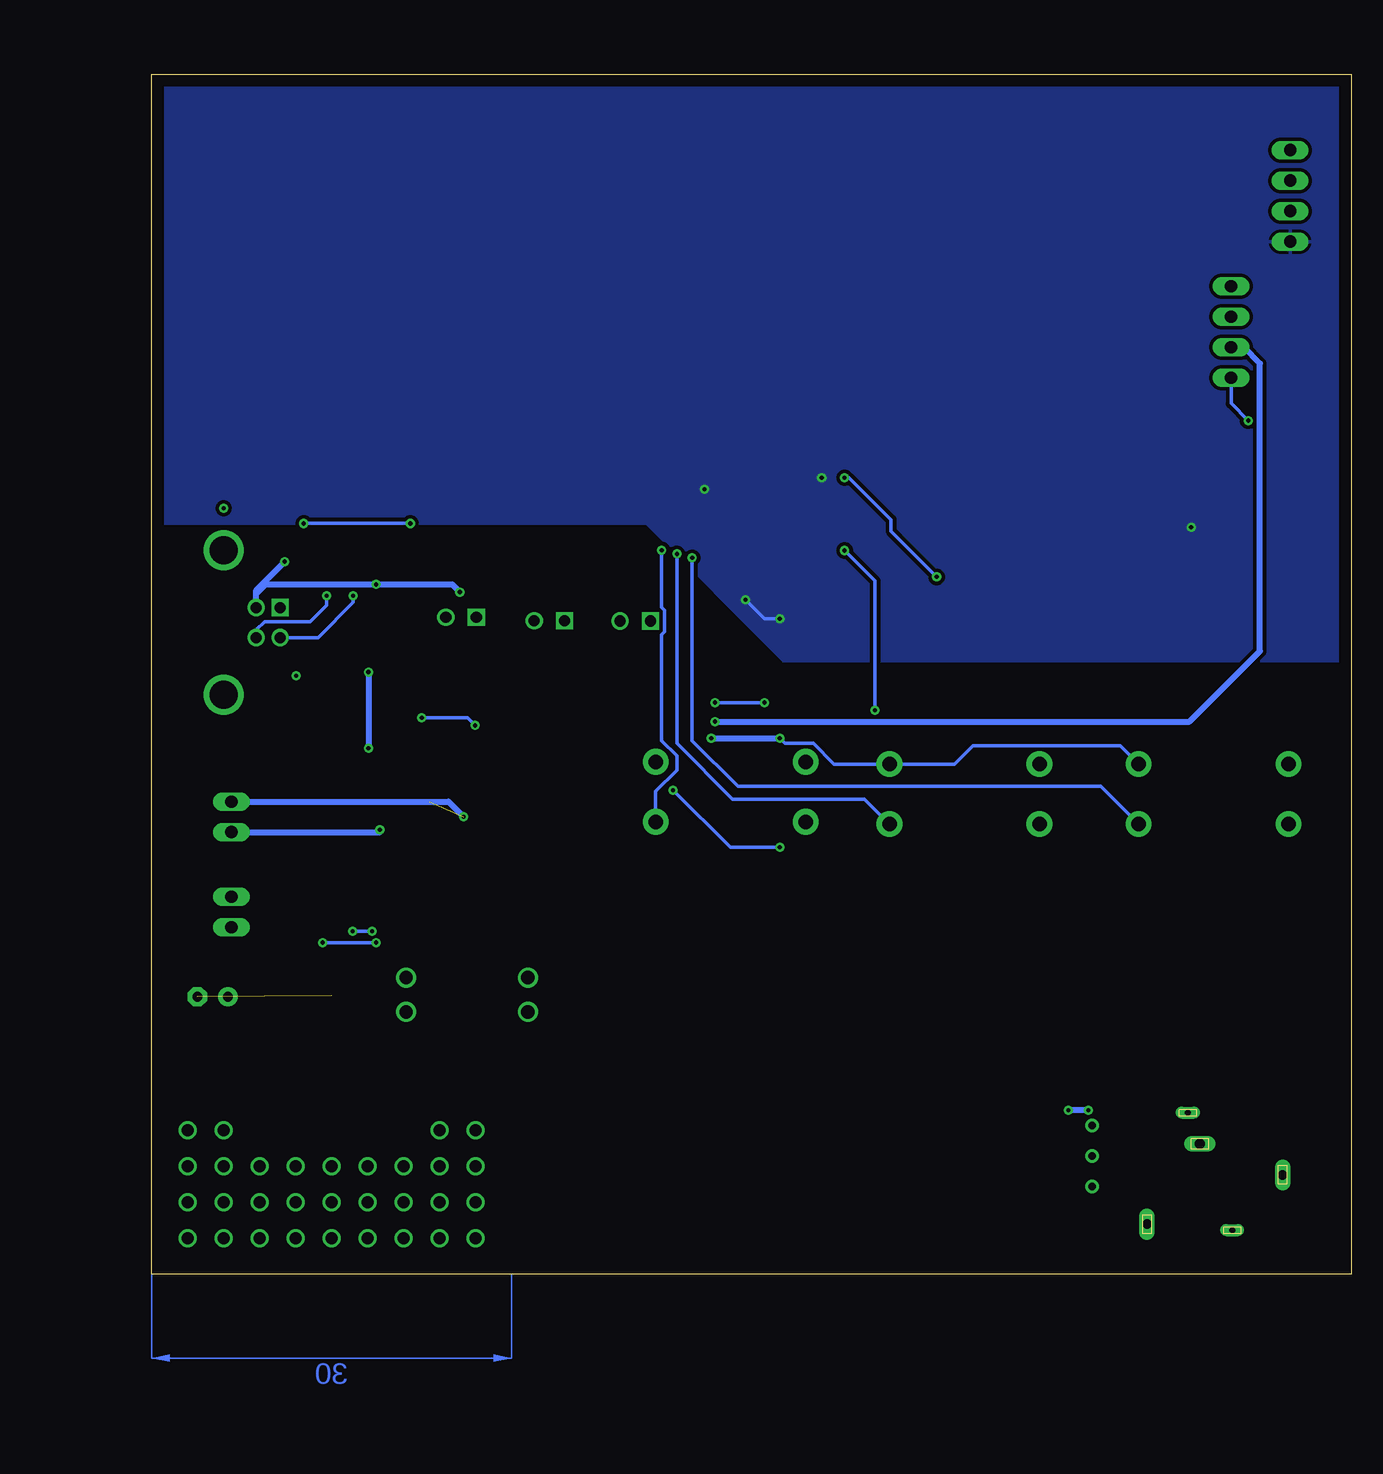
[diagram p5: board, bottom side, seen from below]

Size 100 x 100 mm. Coordinates in mm from the lower left corner, seen from the top.
Outline: 0,0 100,0 100,100 0,100 0,0
Copper layers (1*16): Top 0.035mm / dielectric 1.5mm / Bottom 0.035mm
Design rules "default *": minimum track width 6mil, minimum drill 0.35mm, track to track 6mil, track to pad 6mil, pad to pad 6mil, via to via 6mil, smd to smd 6mil, copper to edge 40mil, drill to drill 6mil, minimum pad ring 10mil, minimum via ring 8mil, stop-mask expansion 4mil, vias tented up to drill 0mil, thermal gap 10mil

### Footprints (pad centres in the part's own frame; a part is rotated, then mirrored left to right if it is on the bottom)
WENZHOU_PJ324M = drill 0.8 long: 1 0,5.4; 3 2.6,-1.5; 4 -4.1,-5.9 | drill 0.5 long: 2 5.2,-2.5; 5 -4.6,1.2
6410-02 = drill 1.016 long: 1 1.27,0; 2 -1.27,0
C0805 = smd 1.3 x 1.5: 1 -0.95,0; 2 0.95,0
B45181A = drill 0.813 pad 1.6: + -1.27,0 | drill 0.813 pad 1.6 octagon: - 1.27,0
SODFL3718X115 = smd 1.115 x 1.361: 1 -1.6,0; 2 1.6,0
DIO_TESD5V0L1UC_RJG = smd 0.41 x 0.56: 1 -0.35,0; 2 0.35,0
DO41-10 = drill 1.118: A 5.08,0; C -5.08,0
1X04 = drill 1.016 long: 1 -3.81,0; 2 -1.27,0; 3 1.27,0; 4 3.81,0
SOT95P280X100-5N = smd 1.05 x 0.55: 1 -1.3,0.95; 2 -1.3,0; 3 -1.3,-0.95; 4 1.3,-0.95; 5 1.3,0.95
SOIC127P600X175-14N = smd 1.968 x 0.599: 1 -2.473,3.81; 2 -2.473,2.54; 3 -2.473,1.27; 4 -2.473,0; 5 -2.473,-1.27; 6 -2.473,-2.54; 7 -2.473,-3.81; 8 2.473,-3.81; 9 2.473,-2.54; 10 2.473,-1.27; 11 2.473,0; 12 2.473,1.27; 13 2.473,2.54; 14 2.473,3.81
DFE2HCAH1R0MJ0L = smd 0.85 x 2.2: 1 -1.025,0; 2 1.025,0
CHIPLED_0805 = smd 1.2 x 1.2: A 0,-1.05; C 0,1.05
LEDRD254W50D500H1060 = drill 0.93 pad 1.4: A 1.27,0 | drill 0.93 pad 1.4 square: C -1.27,0
TACTILE_SWITCH_PTH_12MM = drill 1.2 pad 2.159: 1 6.25,-2.5; 2 -6.25,-2.5; 3 6.25,2.5; 4 -6.25,2.5
3.2X1.5 = smd 1 x 1.8: 1 -1.25,0; 2 1.25,0
SOT23 = smd 1 x 1.4: 1 -0.95,-1.1; 2 0.95,-1.1; 3 0,1.1
R0805 = smd 1.3 x 1.5: 1 -0.95,0; 2 0.95,0
RTRIM3296X = drill 0.61: 1 0,-2.54; 2 0,0; 3 0,2.54
SW_TS-1187A-B-A-B = smd 1 x 0.75: A -3,1.875; B 3,1.875; C -3,-1.875; D 3,-1.875
B1,27 = smd 1.27 x 1.27: TP 0,0
QFP50P900X900X160-48N = smd 1.56 x 0.28: 1 -4.18,2.75; 2 -4.18,2.25; 3 -4.18,1.75; 4 -4.18,1.25; 5 -4.18,0.75; 6 -4.18,0.25; 7 -4.18,-0.25; 8 -4.18,-0.75; 9 -4.18,-1.25; 10 -4.18,-1.75; 11 -4.18,-2.25; 12 -4.18,-2.75; 25 4.18,-2.75; 26 4.18,-2.25; 27 4.18,-1.75; 28 4.18,-1.25; 29 4.18,-0.75; 30 4.18,-0.25; 31 4.18,0.25; 32 4.18,0.75; 33 4.18,1.25; 34 4.18,1.75; 35 4.18,2.25; 36 4.18,2.75 | smd 0.28 x 1.56: 13 -2.75,-4.18; 14 -2.25,-4.18; 15 -1.75,-4.18; 16 -1.25,-4.18; 17 -0.75,-4.18; 18 -0.25,-4.18; 19 0.25,-4.18; 20 0.75,-4.18; 21 1.25,-4.18; 22 1.75,-4.18; 23 2.25,-4.18; 24 2.75,-4.18; 37 2.75,4.18; 38 2.25,4.18; 39 1.75,4.18; 40 1.25,4.18; 41 0.75,4.18; 42 0.25,4.18; 43 -0.25,4.18; 44 -0.75,4.18; 45 -1.25,4.18; 46 -1.75,4.18; 47 -2.25,4.18; 48 -2.75,4.18
SOT95P280X145-5N = smd 1.21 x 0.59: 1 -1.255,0.95; 2 -1.255,0; 3 -1.255,-0.95; 4 1.255,-0.95; 5 1.255,0.95
SOT229P700X180-4N = smd 1.31 x 0.93: 1 -3.345,2.29; 2 -3.345,0; 3 -3.345,-2.29 | smd 1.31 x 3.24: 4 3.345,0
HRP7_ROM-M = smd 0.787 x 1.854: 1 -3.81,-6.172; 2 -2.54,-6.172; 3 -1.27,-6.172; 4 0,-6.172; 5 1.27,-6.172; 6 2.54,-6.172; 7 3.81,-6.172 | smd 7.48 x 7.49: 8 0,1.051
61729-1011BLF = drill 0.92 square: 1 1.25,4.71 | drill 0.92: 2 -1.25,4.71; 3 -1.25,2.71; 4 1.25,2.71 | drill 2.3: SH1 -6.02,0; SH2 6.02,0
CRYSTAL_2-SMD-5X3 = smd 2 x 2.4: 1 -2,0; 2 2,0

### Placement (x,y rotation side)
AUDIO_JACK  11.11,8.26 90 top
BATTERIE  93.34,38.1 90 top
C1  6.03,83.5 0 top
C2  11.11,60.01 90 top
C3  69.77,33.61 90 top
C4  94.91,23.11 0 top
C5  68.75,28.64 270 top
C7  64.14,46.67 90 top
C8  36.2,65.41 0 top
C9  37.47,57.15 0 top
C10  42.86,68.9 270 top
C11  36.51,68.9 270 top
C12  82.87,53.98 0 top
C21  66.36,28.57 90 top
C22  66.99,33.66 90 top
C26  43.18,53.66 90 top
D1  79.38,53.02 90 top
D2  87.31,57.47 270 top
D3  81.28,60.64 90 top
D4  87.31,60.64 90 top
D5  7.94,86.04 180 top
D6  7.94,88.58 180 top
D7  7.94,89.85 180 top
D8  73.7,21.84 180 top
D9  73.7,24.7 180 top
DC-MOTOR  93.34,30.16 90 top
DISPLAY  10,78.5 90 top
IC1  79.69,40.01 90 top
IC4  28.57,8.26 0 top
L1  71.76,28.47 90 top
LED  32.07,58.1 90 top
LED1  87.63,38.42 180 top
LED2  89.53,38.42 180 top
LED_LEFT  59.66,54.42 0 top
LED_MIDDLE  66.83,54.43 0 top
LED_RIGHT  74.19,54.74 0 top
LEFT  11.46,40 0 top
POWER_LED  42.55,50.48 90 top
Q1  39.69,67.94 0 top
Q2  84.77,34.61 90 top
Q3  77.15,43.81 90 top
R1  40.96,53.66 90 top
R2  13.34,60.01 90 top
R3  5.71,73.34 0 top
R4  5.71,71.12 180 top
R5  27.94,58.1 0 top
R6  76.83,40.32 90 top
R7  84.14,40.96 0 top
R8  84.14,38.42 0 top
R9  70.17,45.72 0 top
R10  68.26,41.91 180 top
R11  82.87,51.75 180 top
R12  35.24,61.28 90 top
R13  78.42,60.01 270 top
R25  85.41,60.01 270 top
R26  83.19,60.01 270 top
R27  21.59,3.49 0 top
R28  21.59,9.84 180 top
R29  66.36,46.67 90 top
R30  59.33,58.86 180 top
R31  73.86,59.18 180 top
R32  66.64,59.04 180 top
R33  21.27,36.51 90 top
R35  60.64,38.42 270 top
R36  41.91,36.51 90 top
R37  39.69,70.17 0 top
RESET  6.03,60.96 0 top
RIGHT  32.22,40 0 top
S2  6.03,66.99 0 top
SELECT  51.72,40.18 0 top
ST_LINK  5.08,89.85 270 top
TP1  96.84,46.35 0 top
TP3  64.14,43.5 0 top
TP4  60.01,41.27 0 top
TP5  3.81,13.34 0 top
TP6  24.77,3.17 0 top
U1  47.94,62.55 0 top
U2  72.75,33.49 90 top
U3  60.96,32.07 180 top
U4  85,17 180 top
USB-B  93.98,54.29 90 top
Y1  38.42,61.28 90 top

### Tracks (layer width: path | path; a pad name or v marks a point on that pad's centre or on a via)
+3V3  (via drill 0.35)
  Top 0.203: v50.48,56.2 50.69,56.41 U1.24 | U1.9 43.74,61.28 41.91,61.28 | U1.1 43.76,65.99 v44.13,66.36 44.5,66.73 U1.48 | v53.9,65.41 53.79,65.3 U1.36
  Top 0.305: D5.2 ST_LINK.4 C1.1 3.81,83.5 1.8,81.49 1.8,65.82 2.51,65.12 S2.C S2.D 10.45,65.12 v13.34,62.23 R2.2 | 41.91,61.28 41.39,60.76 41.39,58.94 45.72,54.61 v47.62,54.61 | 61.28,42.23 60.83,42.68 SELECT.3 59.37,41.27 TP4.TP | C26.1 43.59,52.29 POWER_LED.A 45.08,51.97 45.08,52.07 | LEFT.3 18.28,42.5 22.74,38.04 22.74,10.32 24.81,8.26 IC4.4
  Top 0.508: C21.2 66.36,30.8 65.09,32.07 U3.2 63.5,32.07 62.87,32.7 62.87,40.64 61.28,42.23 58.85,44.66 v53.34,44.66 | v47.62,44.66 46.78,44.66 45.08,46.36 45.08,52.07 v47.62,54.61
  Bottom 0.305: v47.62,54.61 48.9,54.61 v50.48,56.2 | v47.62,44.66 47.18,44.22 44.83,44.22 43.11,42.5 RIGHT.3 33.06,42.5 31.53,44.04 19.25,44.04 LEFT.3
  Bottom 0.508: v53.34,44.66 v47.62,44.66
  pour Bottom (isolate 0.305): 0,51.12 47.31,51.12 58.74,62.55 100.01,62.55 100.01,100.01 0,100.01
+5V  (via drill 0.35)
  Top 0.305: TP3.TP 64.14,41.59
  Top 0.508: v53.02,46.04 59.69,46.04 64.14,41.59 64.14,34.53 U3.3 64.38,34.29 66.67,34.29 C22.2 67.03,34.56 C3.2 71.12,35.91 72.53,35.91 U2.4 73.7,36.48 73.04,37.13 73.04,43.2 74.93,45.09 74.93,52.39 78.42,55.88 R13.2
  Bottom 0.508: v53.02,46.04 13.48,46.04 7.6,51.92 7.6,75.87 8.96,77.23 DISPLAY.2
BATTERY_LEVEL  (via drill 0.35)
  Top 0.203: U1.16 46.69,57.15
  Top 0.305: 46.69,57.15 46.69,56.81 48.9,54.61 v48.9,47.62 | v53.02,47.62 C7.2 R29.2
  Bottom 0.305: v48.9,47.62 v53.02,47.62
BOOT0
  Top 0.203: U1.44 47.19,68.58
  Top 0.305: 47.19,68.58 42.43,73.34 R3.2
BUTTON_1  (via drill 0.35)
  Top 0.203: U1.26 53.34,60.3 54.32,60.3
  Top 0.305: R33.2 17.75,37.46 LEFT.1 | 54.32,60.3 v54.93,59.69
  Bottom 0.305: v54.93,59.69 54.93,44.45 51.11,40.64 20.85,40.64 LEFT.1
BUTTON_2  (via drill 0.35)
  Top 0.203: U1.27 53.34,60.8 55.41,60.8
  Top 0.305: RIGHT.1 41.87,37.5 R36.2 | 55.41,60.8 v56.2,60.01
  Bottom 0.305: v56.2,60.01 56.2,44.23 51.55,39.58 40.55,39.58 RIGHT.1
BUTTON_3  (via drill 0.35)
  Top 0.203: U1.28 53.34,61.3 56.49,61.3
  Top 0.305: v57.47,60.33 56.49,61.3 | R35.2 58.18,37.47 SELECT.1
  Bottom 0.305: SELECT.1 57.97,40.22 56.2,41.99 56.2,43.18 57.47,44.45 57.47,53.26 57.22,53.51 57.22,55.33 57.47,55.58 v57.47,60.33
DISPLAY_SCL
  Top 0.203: U1.42 48.19,70.8
  Top 0.305: 48.19,70.8 36.69,82.31 DISPLAY.4
DISPLAY_SDA
  Top 0.203: U1.43 47.69,69.53
  Top 0.305: 47.69,69.53 37.45,79.77 DISPLAY.3
GND  (via drill 0.35)  (2 unrouted)
  Top 0.203: U1.8 45.09,61.8 45.69,62.41 45.69,65.41 | 45.69,65.41 U1.47 45.72,68.58 44.45,69.85 C10.1 | U1.35 51.12,64.8 | 51.12,64.8 46.3,64.8 45.69,65.41 | U1.23 50.19,63.87 51.12,64.8
  Top 0.305: R36.1 v47.62,35.56 | v56.52,40.32 60.01,40.32 60.64,39.69 R35.1 | USB-B.SH1 95.87,48.27 96.84,47.31 TP1.TP | v8.57,71.12 R4.1
  Top 0.508: 93.98,55.23 93.66,55.54 USB-B.4 93.98,58.25 USB-B.SH2 v93.98,63.82 | 93.98,55.23 98.42,50.78 98.42,41.91 | 98.42,41.91 95.89,39.37 BATTERIE.1 | 98.42,41.91 98.42,24.09 97.44,23.11 C4.- | R33.1 21.27,14.29 v21.91,13.65 | 93.98,55.23 USB-B.SH1 89.52,48.27 v87.95,49.85
  Bottom 0.305: v47.62,35.56 51.75,35.56 v56.52,40.32 | DISPLAY.1 10,72.55 v8.57,71.12
  Bottom 0.508: BATTERIE.1 75.25,39.37 v73.98,38.1 | v74.3,56.83 74.93,57.47 v81.28,57.47 90.49,57.47 91.27,56.69 USB-B.4 91.27,57 v88.9,59.37 | v21.91,13.65 v23.58,13.65
  pour Top (isolate 0.305): 99.38,20.64 75.56,20.64 75.56,30.8 99.38,30.8
  pour Top (isolate 0.305): 74.93,26.35 63.82,26.35 63.82,39.05 74.93,39.05
  pour Top (isolate 0.305): 99.38,31.43 75.56,31.43 75.56,44.77 99.38,44.77
  pour Top (isolate 0.305): 2.86,50.16 2.86,33.97 61.91,33.97 61.91,40.32 74.93,40.32 74.93,50.8 76.83,52.7 76.83,60.33 57.47,60.33 57.47,50.16
  pour Top (isolate 0.305): 77.47,61.91 77.47,45.72 89.85,45.72 89.85,61.91
  pour Top (isolate 0.305): 0,0 33.97,0 33.97,14.92 0,14.92
  pour Top (isolate 0.305): 0,100.01 100.01,100.01 100.01,62.55 59.37,62.55 47.94,51.12 0,51.12
LED_LEFT
  Top 0.203: U1.29 53.34,61.8 59.4,61.8
  Top 0.305: LED_LEFT.A 61.39,54.88 61.39,59.8 59.4,61.8
LED_MIDDLE
  Top 0.203: 67.56,62.3 53.34,62.3 U1.30
  Top 0.305: LED_MIDDLE.A 68.69,55.03 68.69,61.16 67.56,62.3
LED_RIGHT
  Top 0.203: U1.31 53.34,62.8 74.05,62.8
  Top 0.305: 74.05,62.8 75.92,60.92 75.92,55.19 LED_RIGHT.A
MOTOR_PWM1
  Top 0.203: U1.18 47.69,57.15
  Top 0.305: D8.A 62.12,21.84 49.85,34.11 49.85,54.61 47.69,56.77 47.69,57.15
MOTOR_PWM2
  Top 0.203: U1.19 48.19,57.15
  Top 0.305: 48.19,57.15 50.48,54.86 50.48,36.02 61.8,24.7 D9.A
MOTORA
  Top 0.508: DC-MOTOR.2 89.85,28.89 87.54,26.58 U4.2
MOTORB
  Top 0.508: DC-MOTOR.1 84.14,31.43 82.46,29.75 U4.6
N$1
  Top 0.508: L1.2 71.8,29.53 U2.1
N$2
  Top 0.305: R5.2 LED.C
N$3
  Top 0.305: R1.1 40.96,51.02 POWER_LED.C
N$4
  Top 0.305: R10.2 67.31,43.5 66.36,44.45 R29.1 R9.1
N$5
  Top 0.305: R3.1 R4.2 3.5,71.12 3.03,70.66 S2.A S2.B
N$6  (via drill 0.35)
  Top 0.305: D8.C 78.78,23.05 80.01,24.28 80.01,26.35 v81.28,27.62 | U4.3 86.27,27.08 v85.72,27.62
  Bottom 0.305: v85.72,27.62 v81.28,27.62
N$8
  Top 0.305: R6.2 76.87,41.3 IC1.5
N$9
  Top 0.305: LED2.C 89.53,36.41 86.78,33.66 Q2.1 84.87,34.66 84.87,36.18 85.09,36.4 R8.2 85.09,37.64 83.65,36.2 80.3,36.2 78.74,37.75 IC1.1
N$10  (via drill 1)
  other vias: 73,3
N$11
  Top 0.305: LED2.A LED1.A 87.63,40.42 87.09,40.96 R7.2
N$12
  Top 0.305: LED1.C 87.63,36.41 86.77,35.56 Q2.2
N$13  (via drill 1)
  other vias: 76,3
N$14  (via drill 0.35)
  Top 0.305: D9.C 78.78,26.29 81.06,28.57 v81.6,28.57 | v83.25,28.57 83.73,28.09 U4.5
  Bottom 0.305: v83.25,28.57 v81.6,28.57
N$15  (via drill 1)
  other vias: 79,3
N$16
  Top 0.305: IC4.6 24.51,5.71 22.93,7.3 R28.3 20.64,6.35 R27.1
N$17  (via drill 1)
  other vias: 82,3
N$18  (via drill 1)
  other vias: 85,3
N$19
  Top 0.305: LED_LEFT.C 58.4,58.88 R30.2
N$20
  Top 0.305: LED_RIGHT.C 72.92,59.17 R31.2
N$21  (via drill 1)
  other vias: 88,3
N$22  (via drill 1)
  other vias: 91,3
N$23
  Top 0.305: LED_MIDDLE.C 65.56,58.91 R32.2
N$24  (via drill 1)
  other vias: 94,3
N$25  (via drill 1)
  other vias: 97,3
N$26  (via drill 1)
  other vias: 97,6
N$27  (via drill 1)
  other vias: 94,6
N$28  (via drill 1)
  other vias: 91,6
N$29  (via drill 0.35)
  Top 0.305: v85.41,56.52 R25.2
  Bottom 0.305: USB-B.3 91.27,53.68 90.58,54.37 86.78,54.37 85.41,55.74 v85.41,56.52
N$30  (via drill 0.35)
  Top 0.305: R26.2 v83.19,56.52
  Bottom 0.305: USB-B.2 86.11,53.04 83.19,55.97 v83.19,56.52
N$31  (via drill 1)
  other vias: 91,9
N$32  (via drill 1)
  other vias: 94,9
N$33  (via drill 1)
  other vias: 97,9
N$34  (via drill 1)
  other vias: 88,9
N$35  (via drill 1)
  other vias: 85,9
N$36  (via drill 1)
  other vias: 82,9
N$37  (via drill 1)
  other vias: 79,9
N$38  (via drill 1)
  other vias: 76,9
N$39  (via drill 1)
  other vias: 73,9
N$40  (via drill 1)
  other vias: 73,6
N$41  (via drill 1)
  other vias: 76,6
N$42  (via drill 1)
  other vias: 79,6
N$43  (via drill 1)
  other vias: 82,6
N$44  (via drill 1)
  other vias: 85,6
N$45  (via drill 1)
  other vias: 88,6
N$46  (via drill 1)
  other vias: 73,12
N$47  (via drill 1)
  other vias: 76,12
N$48  (via drill 1)
  other vias: 97,12
N$49  (via drill 1)
  other vias: 94,12
OSC32IN
  Top 0.203: U1.3 42.7,64.3 40.94,66.06 Q1.2
  Top 0.305: C10.2 Q1.2 40.94,69.87 R37.2
OSC32OUT
  Top 0.203: U1.4 41.31,63.8 38.44,66.67 Q1.1
  Top 0.305: C11.2 Q1.1 | Q1.1 | R37.1 38.44,69.86 Q1.1
OSCIN
  Top 0.203: U1.5 38.44,63.3 Y1.2
  Top 0.305: R12.2 35.24,62.86 35.66,63.28 Y1.2 38.42,64.77 37.78,65.41 C8.2
OSCOUT
  Top 0.203: Y1.1 38.42,60.33 40.89,62.8 U1.6
  Top 0.305: R12.1 35.24,59.69 35.66,59.28 Y1.1 C9.2
PAD
  pour Top: 100,0 70,0 70,20 100,20
PC13  (via drill 0.35)
  Top 0.203: U1.2 42.84,64.8 42.55,65.09 42.55,66.04 v42.23,66.36
  Top 0.305: LED.A v34.55,58.1
  Bottom 0.305: v34.55,58.1 38.36,61.91 38.36,62.87 41.85,66.36 v42.23,66.36
RESET
  Top 0.203: 42.55,62.3 U1.7
  Top 0.305: 42.55,62.3 41.34,62.3 40.32,61.28 40.32,57.01 39.25,55.94 25.97,55.94 22.86,59.06 R2.1 C2.1 9.06,59.06 RESET.D RESET.C
SIGNAL_IN
  Top 0.305: AUDIO_JACK.5 11.28,3.65 16.19,8.57 17.46,8.57 | IC4.5 24.45,6.99 22.86,8.57 17.46,8.57 | 17.46,8.57 13.61,12.42 AUDIO_JACK.2 13.49,13.34 TP5.TP
SIGNAL_OPAMP  (via drill 0.35)
  Top 0.203: U1.11 42.55,60.3
  Top 0.305: 42.55,60.3 v42.23,60.3 | v39.69,46.97 39.69,45.92 40.32,45.28 40.32,41.52 36.83,38.03 36.83,3.49 35.78,2.44 27.3,2.44 26.14,3.6 26.1,3.64 IC4.7 23.49,4.45 R27.2 24.45,3.49 TP6.TP
  Bottom 0.305: v42.23,60.3 39.69,57.76 v39.69,46.97
SWDCLK
  Top 0.203: 50.69,69.53 U1.37
  Top 0.305: ST_LINK.2 6.35,89.85 D7.2 7.59,90.49 8.86,91.76 28.47,91.76 50.69,69.53
SWDIO
  Top 0.203: U1.34 53.98,64.3
  Top 0.305: D6.2 ST_LINK.3 3.81,88.58 3.1,89.29 3.1,91.63 3.81,92.34 30.65,92.34 54.74,68.25 54.74,65.06 53.98,64.3
USB+  (via drill 0.35)
  Top 0.203: U1.33 52.12,63.82 83.41,63.82
  Top 0.305: 83.41,63.82 85.41,61.82 R25.1 87.28,60.96 D4.2 v87.31,62.55 | R13.1 v78.42,62.55
  Bottom 0.305: v78.42,62.55 v87.31,62.55
USB-
  Top 0.203: U1.32 53.34,63.3 79.89,63.3
  Top 0.305: D3.2 81.31,60.96 R26.1 82.23,60.96 79.89,63.3
VBAT  (via drill 0.35)
  Top 0.305: R9.2 v73.03,45.72 | Q3.2 78.25,45.57 v77.47,46.35
  Top 0.508: U4.1 88.87,23.11 C4.+ 96.23,25.71 96.23,33.95 BATTERIE.2 93.25,36.83 90.81,39.28 90.81,40.19 86.23,44.77 Q3.2 | v80.96,37.03 80.64,37.35 IC1.3
  Bottom 0.305: v73.03,45.72 73.66,46.35 v77.47,46.35
  Bottom 0.508: BATTERIE.2 80.96,36.83 v80.96,37.03
VBUS  (via drill 0.35)
  Top 0.305: R8.1 R7.1 82.84,41.3 IC1.4 | IC1.4 80.64,42.23
  Top 0.508: 80.64,42.23 80.01,42.87 Q3.1 80.97,42.87 v81.92,43.81 | IC1.4 | v81.92,50.16 R11.2 C12.1 81.27,54.62 D1.2 80.3,55.54 87.95,55.54 | USB-B.1 87.95,55.54 | D2.2 87.31,56.18 87.95,55.54
  Bottom 0.508: v81.92,50.16 v81.92,43.81
VIN
  Top 0.508: D1.1 77.47,49.52 77.47,48.26 76.05,46.84 Q3.3 75.53,43.29 75.53,29.67 73.3,27.45 L1.1 68.99,27.45 C5.2
(copper drawn outside any net)
  shapes: Bottom area x1, Top area x7

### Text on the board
tNames: Gabriel Unterweger / 5BEL
tDocu: BATTERY | MOTOR

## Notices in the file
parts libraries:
crystal-geyer_V1_0: Copyright: Geyer-Electronic
SparkFun-Switches: Licensing: Creative Commons ShareAlike 4.0 International - https://creativecommons.org/licenses/by-sa/4.0
